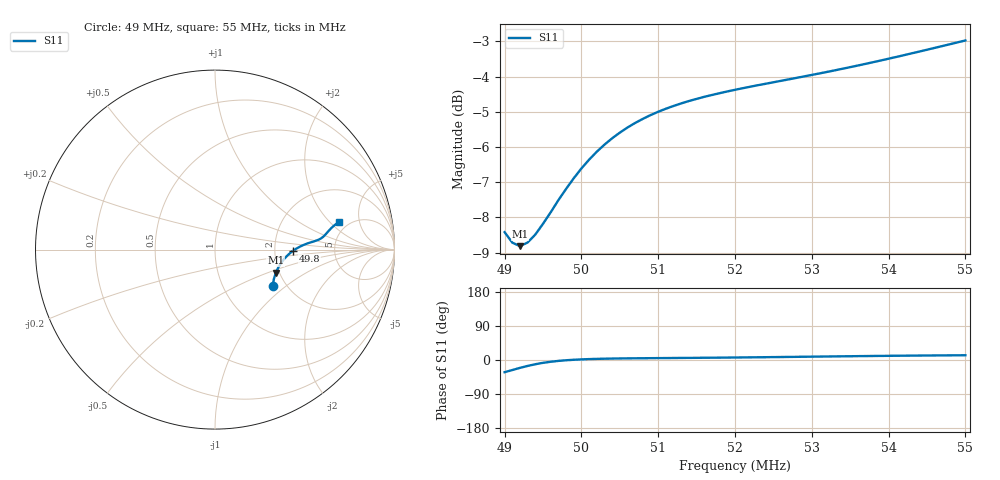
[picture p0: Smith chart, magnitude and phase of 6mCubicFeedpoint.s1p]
# MHz S RI R 50
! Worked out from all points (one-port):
!   61 points, 49 MHz to 55 MHz, reference 50 ohm
!   lowest |S11| = -8.8 dB at 49.2 MHz (marker M1), VSWR 2.14, Z = 95.7 - j28.3 ohm
!   |S11| at or under -10 dB: nowhere
!   S11 on the Smith chart (normalised r, x): 49 MHz: 1.71, -0.81; 49.8 MHz: 2.55, -0.03; 55 MHz: 4.21, +2.61
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49  0.3213 -0.2018
49.1  0.3281 -0.1636
49.2  0.3388 -0.1286
49.3  0.3532 -0.0988
49.4  0.3693 -0.073
49.5  0.3866 -0.0508
49.6  0.4035 -0.0327
49.7  0.4208 -0.0174
49.8  0.4369 -0.00528
49.9  0.4524 0.00481
50  0.467 0.0132
50.1  0.4804 0.02
50.2  0.4928 0.0256
50.3  0.5041 0.0301
50.4  0.5145 0.0341
50.5  0.5239 0.0373
50.7  0.5405 0.0425
50.9  0.5543 0.0469
51.1  0.5657 0.0508
51.3  0.5754 0.0546
51.6  0.5874 0.0605
52  0.6002 0.0694
52.4  0.6111 0.0796
52.8  0.6216 0.0911
53.5  0.6409 0.1125
53.9  0.6532 0.1247
54.3  0.6669 0.1363
55  0.6931 0.1537
